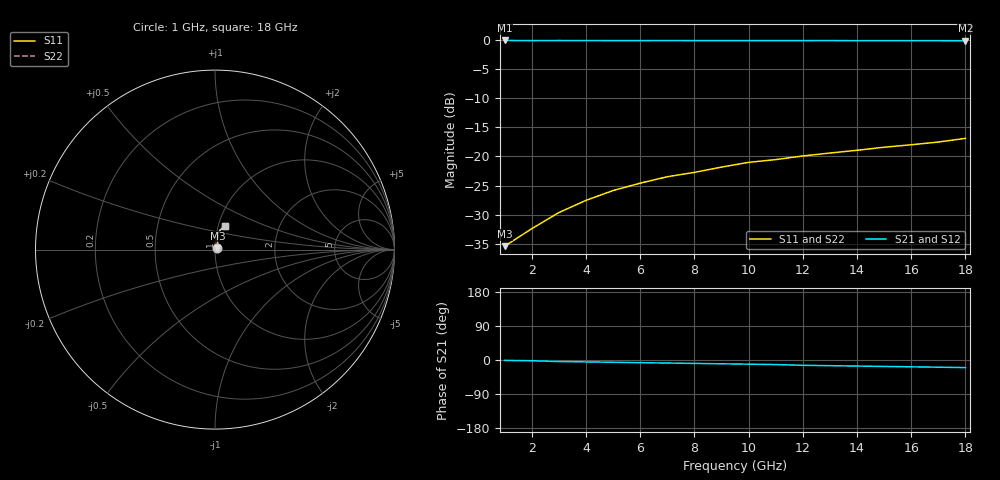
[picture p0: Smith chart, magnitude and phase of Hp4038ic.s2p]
!HPND-4038 beam lead PIN diode
!Series configuration S-parameters If= 10 mA.  Last updated 10/3/97
# mhz s ma r 50
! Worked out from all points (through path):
!   18 points, 1 GHz to 18 GHz, reference 50 ohm
!   highest |S21| = -0.10 dB at 1 GHz (marker M1); lowest = -0.1 dB at 18 GHz (marker M2)
!   group delay of S21, straight-line fit = 3.09 ps
!   lowest |S11| = -35.4 dB at 1 GHz (marker M3), VSWR 1.03, Z = 51.4 + j1 ohm
!   |S11| at or under -10 dB: start of sweep to end of sweep
!   |S22| runs from -35.4 to -16.9 dB; largest |S21 - S12| = 0
1000  0.017 35.0  0.989 -1.0  0.989 -1.0  0.017 35.0
2000  0.024 56.0  0.986 -2.0  0.986 -2.0  0.024 56.0
3000  0.033 66.0  0.988 -4.0  0.988 -4.0  0.033 66.0
4000  0.042 70.0  0.987 -5.0  0.987 -5.0  0.042 70.0
5000  0.051 75.0  0.986 -6.0  0.986 -6.0  0.051 75.0
6000  0.059 77.0  0.986 -7.0  0.986 -7.0  0.059 77.0
7000  0.067 78.0  0.987 -8.0  0.987 -8.0  0.067 78.0
8000  0.073 78.0  0.986 -9.0  0.986 -9.0  0.073 78.0
9000  0.081 78.0  0.986 -10.0  0.986 -10.0  0.081 78.0
10000  0.089 79.0  0.986 -11.0  0.986 -11.0  0.089 79.0
11000  0.094 79.0  0.986 -12.0  0.986 -12.0  0.094 79.0
12000  0.101 77.0  0.986 -14.0  0.986 -14.0  0.101 77.0
13000  0.107 76.0  0.987 -15.0  0.987 -15.0  0.107 76.0
14000  0.113 75.0  0.984 -16.0  0.984 -16.0  0.113 75.0
15000  0.12 73.0  0.985 -17.0  0.985 -17.0  0.12 73.0
16000  0.126 72.0  0.984 -18.0  0.984 -18.0  0.126 72.0
17000  0.133 69.0  0.984 -19.0  0.984 -19.0  0.133 69.0
18000  0.143 67.0  0.983 -20.0  0.983 -20.0  0.143 67.0
